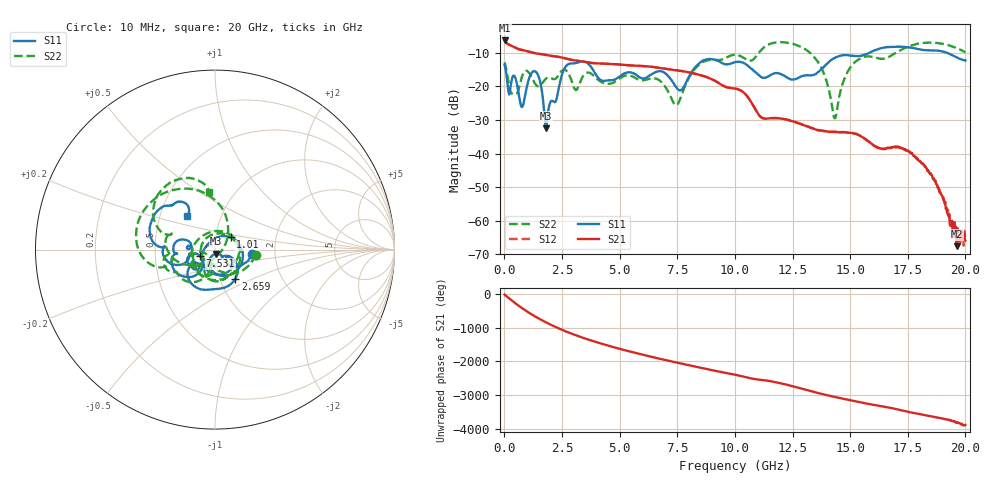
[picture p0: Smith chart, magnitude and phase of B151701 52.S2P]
!  2-Port S-parameters saved by WinCal
! VAR MeasName=S-Parameters (CALIBRATED_DATA) read from VNA (N5244A)
! VAR MeasDate=2015-12-24 19:15:40
! VAR NAME=B151701 52
! VAR FILENAME=B151701 52.S2P
! VAR DATE=2015-12-24 19:15:40
! VAR PHYS_PORTS=1,3
# Hz S DB R 50
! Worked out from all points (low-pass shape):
!   801 points, 10 MHz to 20 GHz, reference 50 ohm
!   highest |S21| = -6.33 dB at 10 MHz (marker M1); lowest = -67.6 dB at 19.63 GHz (marker M2)
!   |S21| within 3 dB of the highest: start of sweep to 882.9 MHz
!   lowest |S11| = -32.5 dB at 1.809 GHz (marker M3), VSWR 1.05, Z = 50.6 - j2.32 ohm
!   |S11| at or under -10 dB: start of sweep to 15.83 GHz; 19.19 GHz to end of sweep
!   |S22| runs from -29.5 to -6.8 dB; largest |S21 - S12| = 0.0011
!   S11 on the Smith chart (normalised r, x): 10 MHz: 1.53, -0.07; 1.01 GHz: 1.18, +0.16; 2.659 GHz: 1.18, -0.40; 7.531 GHz: 0.84, -0.06; 20 GHz: 0.69, +0.27
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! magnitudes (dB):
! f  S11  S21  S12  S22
! 10 MHz  -13.6  -6.3  -6.3  -12.8
! 209.9 MHz  -22.4  -7.6  -7.6  -20.1
! 384.8 MHz  -16.8  -8.1  -8.1  -21.8
! 759.6 MHz  -26.2  -9.2  -9.1  -17.2
! 1.01 GHz  -19.1  -9.6  -9.6  -15.5
! 1.434 GHz  -16.3  -10.2  -10.2  -19.9
! 1.809 GHz  -32.5  -10.6  -10.6  -17.7
! 2.659 GHz  -14.1  -11.7  -11.7  -15.1
! 3.358 GHz  -12.6  -12.6  -12.6  -17.6
! 4.283 GHz  -18.4  -13.2  -13.2  -18.9
! 6.682 GHz  -15.5  -14.4  -14.4  -18.0
! 7.531 GHz  -20.9  -15.3  -15.2  -25.1
! 8.431 GHz  -13.2  -16.5  -16.5  -13.6
! 10.01 GHz  -12.8  -20.7  -20.6  -10.6
! 11.18 GHz  -17.3  -29.4  -29.4  -8.9
! 13.35 GHz  -16.7  -32.4  -32.4  -10.6
! 14.33 GHz  -11.5  -33.5  -33.6  -29.5
! 15.15 GHz  -11.0  -34.0  -34.1  -13.1
! 16.68 GHz  -8.3  -38.3  -38.3  -11.2
! 18.23 GHz  -9.2  -43.6  -43.6  -7.0
! 19.63 GHz  -11.4  -67.6  -64.6  -8.6
! 20 GHz  -12.3  -65.9  -64.6  -9.9
